VAR_GLOBAL CONSTANT
	// Sampling
	cOversamples 		: UDINT 	:= 10;											// number of oversamples
	cSampleRate			: LREAL		:= 10000.0;										// Sample rate of input signal
	
	// Resolution
	cFFTLength			: UDINT		:= 2048;										// length of FFT
	cResolution			: LREAL		:= cSampleRate / cFFTLength;					// Reslution in frequency domain
	cDecimationFactor	: UDINT		:= 16;											// FFT decimation factor, power of 2
	
	// Signal generation
	cSetFrequency		: LREAL 	:= 42 * cResolution;							// Frequency of generated signal in Hz
	cSetFrequencyExt	: LREAL 	:= (42 + 5 * cDecimationFactor) * cResolution;	// Frequency of generated signal in Hz
	cSetAmplitude		: LREAL 	:= 13;											// peak amplitude of sin signal in Volts	
    cDC					: LREAL 	:= 7;       									// Amplitude of DC in Volts
	
	// Streams
	cBufferLength		: UDINT		:= cFFTLength;	     							// attention: needs to be equal to cFFTLength (no overlap)	
	cFFTResult 			: UDINT 	:= cFFTLength / 2 + 1;							// length of one sided spectrum
	cZoomFFTResult		: UDINT 	:= cFFTLength / (2 * cDecimationFactor) + 1;	// length of one sided zoomed spectrum

	// Scope
	cDiameter			: LREAL		:= cFFTLength / (2 * cDecimationFactor);
	cBandwidth			: LREAL		:= cDiameter * cResolution;
	cLower				: LREAL		:= cSetFrequency - (cDiameter / 2) * cResolution;
	cUpper				: LREAL		:= cSetFrequency + (cDiameter / 2) * cResolution;	
	
END_VAR
